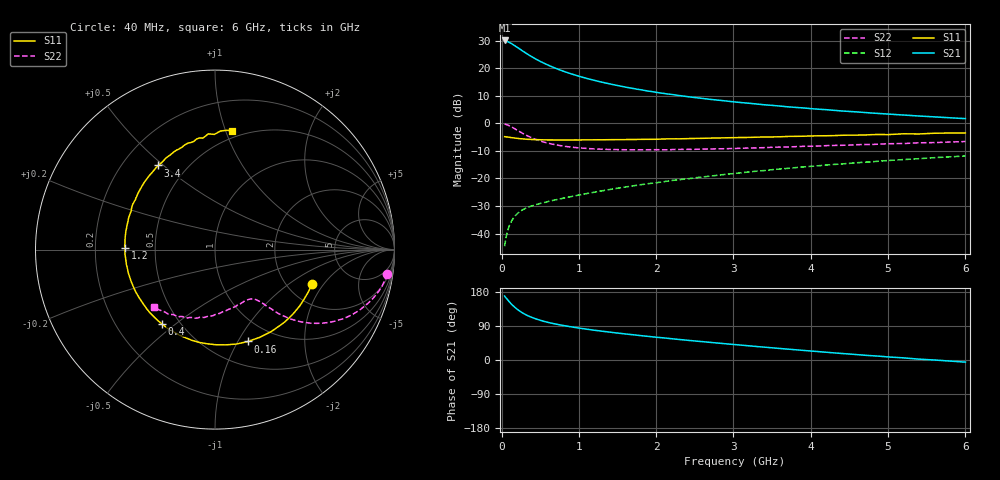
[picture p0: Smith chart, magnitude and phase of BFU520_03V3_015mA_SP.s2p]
! Filename:  P:\Prog\Test\Noise\ATS_data\Testdata_Net\03 Spar\BFU520_APG2013_37_A05_03p3V_015mA_SP_CM01_D.s2p
! Date/Time: Fri 26/Apr/2013 13:00:07
! BFU520_APG2013_37_A05_03p3V_1to20mA_SP_CM01_Bias7_R.s2p
! MDIF S-parameter v. bias file
! BFU520_APG2013_37_A05_03p3V_1to20mA_SP_CM01
! Date/time Tue Apr 23 14:11:50 2013
! VAR V_out= 3.3000
! VAR I_out= 15.0000
! VAR V_in= 0.8531
! VAR I_in= 0.1787
! Device data file deembeded for feedlines and parallel
! Original file: \03 Spar\BFU520_APG2013_37_A05_03p3V_015mA_SP_CM01_R.s2p
! Feed-files: PR047V01_250413_Feed1.s2p, PR047V01_250413_Feed2.s2p
! Parallel-file: PR047V01_250413_Par.s2p
# MHz S MA R 50
!  Freq-MHz  S11-mag  S11-arg  S21-mag  S21-arg  S12-mag  S12-arg  S22-mag  S22-arg
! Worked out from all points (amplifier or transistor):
!   98 points, 40 MHz to 6 GHz, reference 50 ohm
!   highest |S21| = 30.1 dB at 40 MHz (marker M1)
!   |S21| within 3 dB of that: start of sweep to 230.3 MHz
!   unconditionally stable (mu >= 1): 1.346 GHz to 3.47 GHz
!   at 300 MHz: K = 0.42, MSG = 28.4 dB, |S12| = -31.0 dB
!   at 1.6 GHz: K = 1.04, MAG = 16.9 dB, |S12| = -23.1 dB
!   at 6 GHz: K = 0.82, MSG = 6.8 dB, |S12| = -11.8 dB
!   S11 on the Smith chart (normalised r, x): 40 MHz: 2.69, -1.56; 160 MHz: 0.76, -1.10; 400 MHz: 0.40, -0.45; 1.2 GHz: 0.33, +0.01; 3.4 GHz: 0.35, +0.48; 6 GHz: 0.44, +1.05
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40  0.574 -19.8  31.85 168.9  0.005919 81.9  0.9696 -8.1
50  0.5708 -24.6  31.73 165.6  0.007248 80.2  0.9619 -10.1
90  0.5618 -42.7  29.8 156.1  0.0125 73.4  0.9177 -17.6
120  0.554 -55.4  28.42 149.3  0.01587 68.8  0.8746 -22.6
160  0.5435 -70.4  26.16 141.3  0.01968 63.7  0.8146 -28.1
180  0.5397 -77.1  25.11 137.8  0.0213 61.7  0.7836 -30.4
220  0.5303 -89.3  23.08 131.2  0.02404 58.4  0.7261 -34.4
280  0.5217 -104.2  20.21 123.3  0.02729 54.9  0.6507 -38.7
340  0.513 -116.1  17.85 117.0  0.02982 52.7  0.5896 -41.7
400  0.5089 -125.8  15.88 111.8  0.032 51.6  0.5403 -43.7
500  0.504 -138.4  13.31 105.0  0.0352 50.9  0.48 -45.9
650  0.5006 -152.2  10.64 97.0  0.03958 51.5  0.4216 -47.8
800  0.4994 -162.1  8.817 91.0  0.04397 52.8  0.3867 -49.1
1050  0.5007 -174.9  6.839 82.8  0.05159 55.0  0.3548 -51.5
1200  0.5022 179.1  6.019 78.6  0.05639 56.1  0.3441 -53.1
1600  0.5077 165.7  4.551 68.8  0.06991 57.8  0.3322 -58.5
2050  0.5173 154.2  3.563 59.2  0.08547 58.5  0.3321 -66.0
3100  0.5531 130.3  2.38 39.2  0.1269 56.5  0.3533 -84.7
3400  0.5657 124.0  2.169 33.9  0.1394 55.0  0.3626 -90.2
4100  0.594 111.3  1.803 22.1  0.1702 51.0  0.3873 -102.9
5200  0.6461 93.3  1.414 5.6  0.2201 42.9  0.43 -122.6
6000  0.67 81.8  1.218 -5.7  0.256 35.9  0.4675 -136.6
